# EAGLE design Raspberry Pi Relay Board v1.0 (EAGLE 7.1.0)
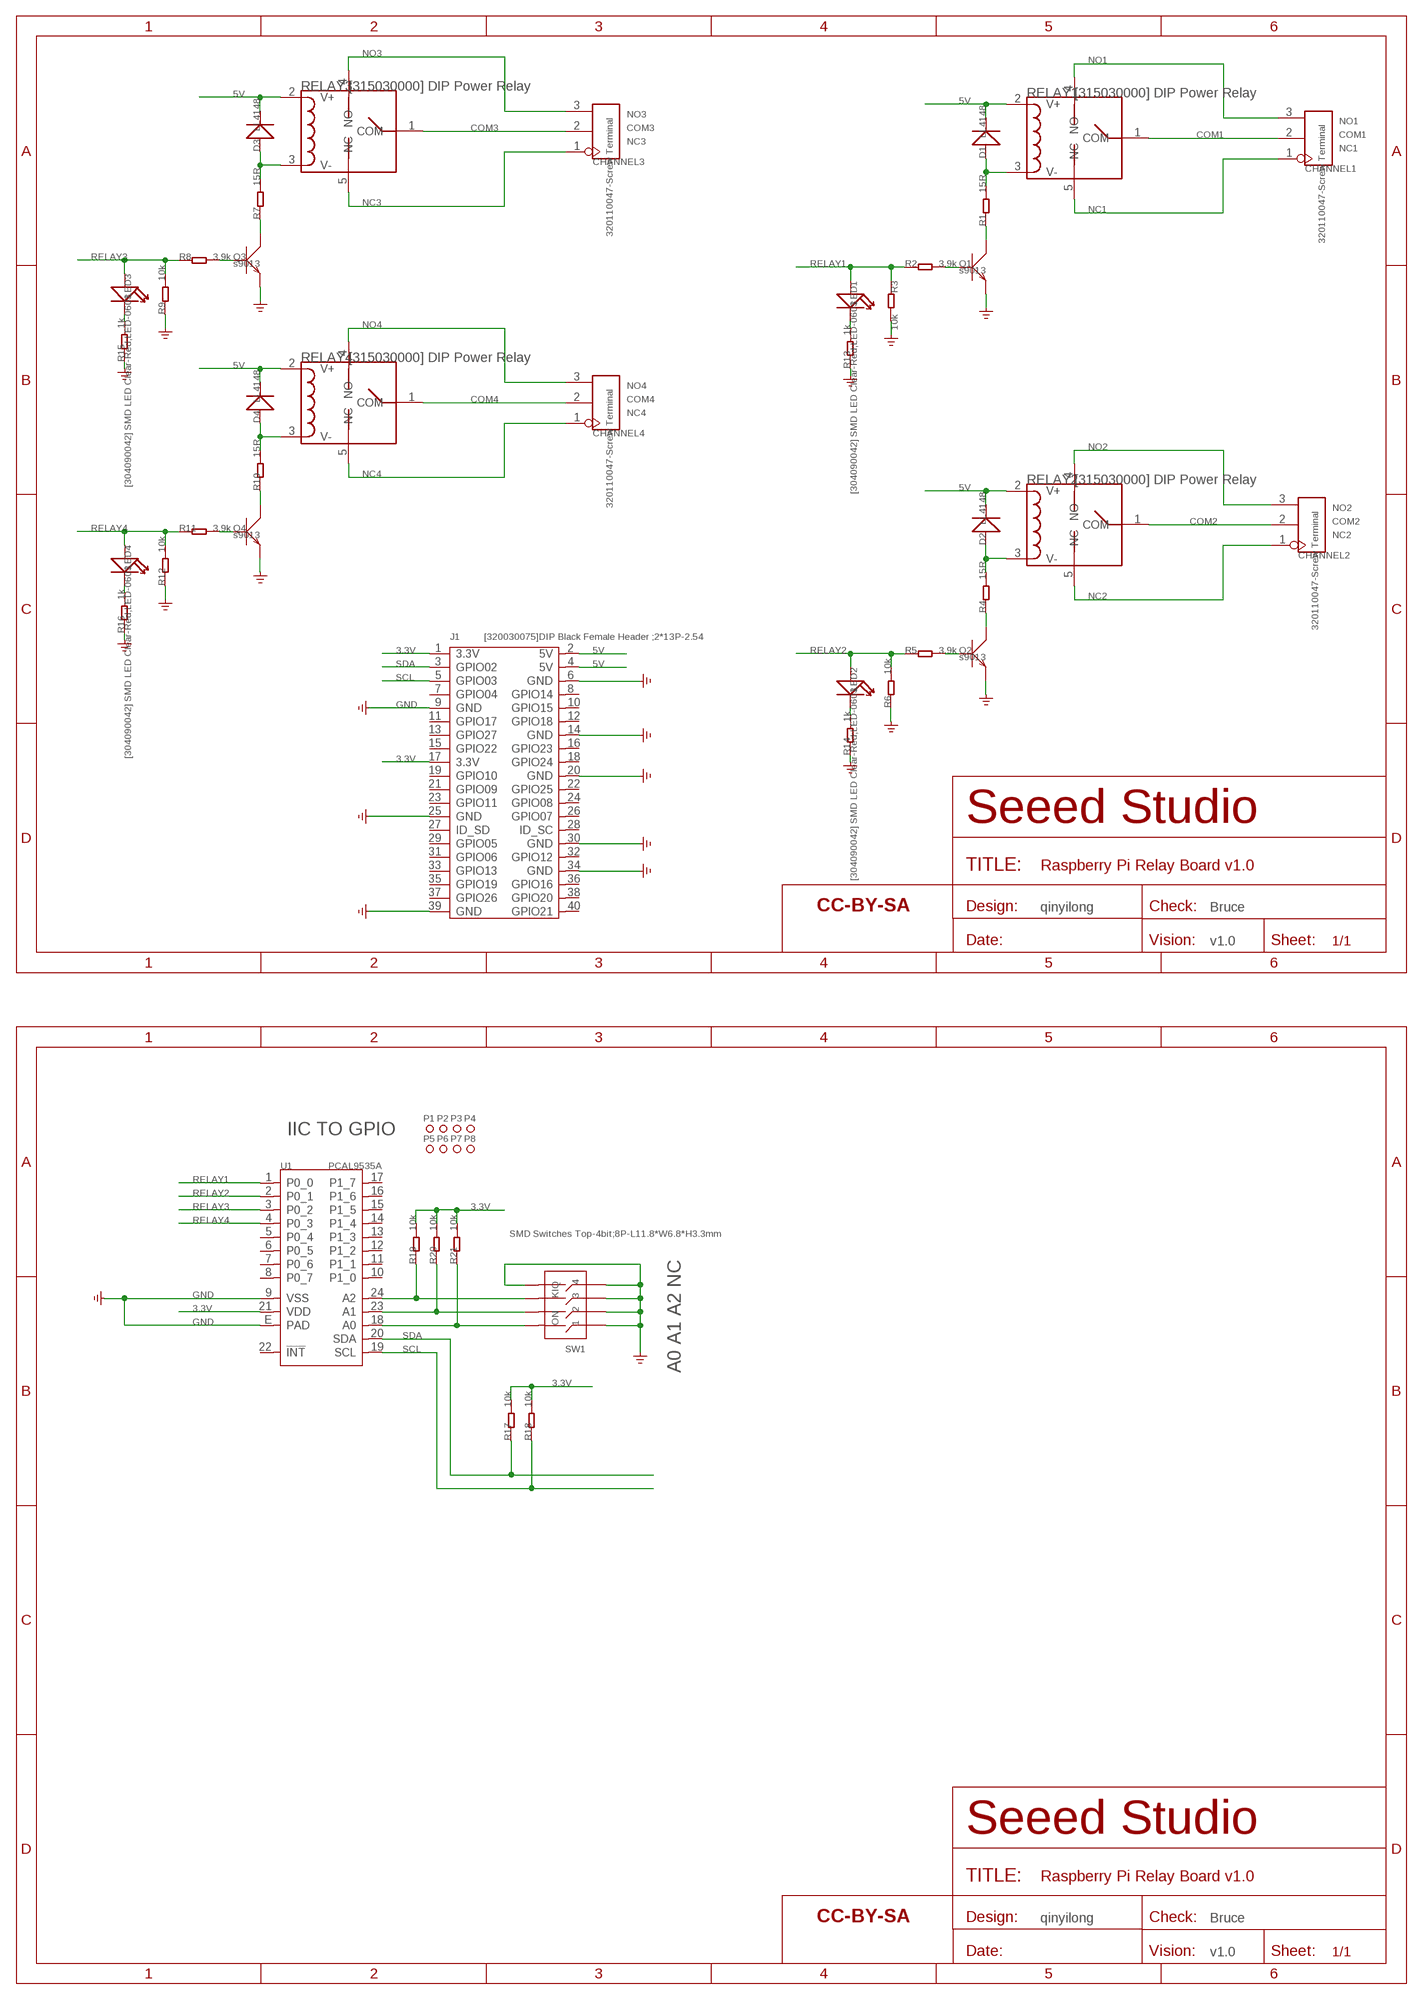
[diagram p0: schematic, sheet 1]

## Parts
CHANNEL1  320110047-Screw Terminal  SCREW-TERMINAL-3P'3.5'  [3P-3.5]
CHANNEL2  320110047-Screw Terminal  SCREW-TERMINAL-3P'3.5'  [3P-3.5]
CHANNEL3  320110047-Screw Terminal  SCREW-TERMINAL-3P'3.5'  [3P-3.5]
CHANNEL4  320110047-Screw Terminal  SCREW-TERMINAL-3P'3.5'  [3P-3.5]
D1  LL4148  D'1N4148-SMD'  [LL-34]
D2  LL4148  D'1N4148-SMD'  [LL-34]
D3  LL4148  D'1N4148-SMD'  [LL-34]
D4  LL4148  D'1N4148-SMD'  [LL-34]
J1  [320030075]DIP Black Female Header ;2*13P-2.54  HEADER-2X20P  [2X20P-2.54-65/35MIL]
LED1  [304090042] SMD LED Clear-Red;LED-0603  LED'0603'  [LED-0603]
LED2  [304090042] SMD LED Clear-Red;LED-0603  LED'0603'  [LED-0603]
LED3  [304090042] SMD LED Clear-Red;LED-0603  LED'0603'  [LED-0603]
LED4  [304090042] SMD LED Clear-Red;LED-0603  LED'0603'  [LED-0603]
P1  PAD-MARK'ANNULAR'  [ROUND-MARK-1.0]
P2  PAD-MARK'ANNULAR'  [ROUND-MARK-1.0]
P3  PAD-MARK'ANNULAR'  [ROUND-MARK-1.0]
P4  PAD-MARK'ANNULAR'  [ROUND-MARK-1.0]
P5  PAD-MARK'ANNULAR'  [ROUND-MARK-1.0]
P6  PAD-MARK'ANNULAR'  [ROUND-MARK-1.0]
P7  PAD-MARK'ANNULAR'  [ROUND-MARK-1.0]
P8  PAD-MARK'ANNULAR'  [ROUND-MARK-1.0]
Q1  s9013  TRANSISTOR-NPN-SOT23  [SOT23]
Q2  s9013  TRANSISTOR-NPN-SOT23  [SOT23]
Q3  s9013  TRANSISTOR-NPN-SOT23  [SOT23]
Q4  s9013  TRANSISTOR-NPN-SOT23  [SOT23]
R1  15R  R-0603  [R0603]
R2  3.9k  R-0603  [R0603]
R3  10k  R-0603  [R0603]
R4  15R  R-0603  [R0603]
R5  3.9k  R-0603  [R0603]
R6  10k  R-0603  [R0603]
R7  15R  R-0603  [R0603]
R8  3.9k  R-0603  [R0603]
R9  10k  R-0603  [R0603]
R10  15R  R-0603  [R0603]
R11  3.9k  R-0603  [R0603]
R12  10k  R-0603  [R0603]
R13  1k  R-0603  [R0603]
R14  1k  R-0603  [R0603]
R15  1k  R-0603  [R0603]
R16  1k  R-0603  [R0603]
R17  10k  R-0603  [R0603]
R18  10k  R-0603  [R0603]
R19  10k  R-0603  [R0603]
R20  10k  R-0603  [R0603]
R21  10k  R-0603  [R0603]
RELAY1  [315030000] DIP Power Relay  RELAY-HLS8L-DC5V-S-C  [5P-19.0X15.5X15.8H]
RELAY2  [315030000] DIP Power Relay  RELAY-HLS8L-DC5V-S-C  [5P-19.0X15.5X15.8H]
RELAY3  [315030000] DIP Power Relay  RELAY-HLS8L-DC5V-S-C  [5P-19.0X15.5X15.8H]
RELAY4  [315030000] DIP Power Relay  RELAY-HLS8L-DC5V-S-C  [5P-19.0X15.5X15.8H]
SW1  SMD Switches Top-4bit;8P-L11.8*W6.8*H3.3mm  SWITCHES-8P'KM-04'  [8P-SMD-L11.8*W6.8*H3.3MM]
U1  PCAL9535A  [QFN24]
U$23  SEEEDSTUDIO-OPEN-SCH-FRAME  [SEEEDSTUDIO-PCB-FRAME]
U$24  SEEEDSTUDIO-OPEN-SCH-FRAME  [SEEEDSTUDIO-PCB-FRAME]

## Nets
3.3V: J1.1(3.3V) J1.17(3.3V) R17.2 R18.2 R19.2 R20.2 R21.2 U1.21(VDD)
5V: D1.C(-) D2.C(-) D3.C(-) D4.C(-) J1.2(5V) J1.4(5V) RELAY1.2(V+) RELAY2.2(V+) RELAY3.2(V+) RELAY4.2(V+)
COM1: CHANNEL1.2 RELAY1.1(COM)
COM2: CHANNEL2.2 RELAY2.1(COM)
COM3: CHANNEL3.2 RELAY3.1(COM)
COM4: CHANNEL4.2 RELAY4.1(COM)
GND: J1.6(GND) J1.9(GND) J1.14(GND) J1.20(GND) J1.25(GND) J1.30(GND) J1.34(GND) J1.39(GND) Q1.2(E) Q2.2(E) Q3.2(E) Q4.2(E) R3.2 R6.1 R9.1 R12.1 R13.1 R14.1 R15.1 R16.1 SW1.1 SW1.2 SW1.3 SW1.4 SW1.5 U1.9(VSS) U1.E(PAD) ; supply symbol labelled GND_POWER
N$1: D2.A(+) R4.2 RELAY2.3(V-)
N$2: D3.A(+) R7.2 RELAY3.3(V-)
N$3: D4.A(+) R10.2 RELAY4.3(V-)
N$4: Q1.3(C) R1.1
N$5: Q2.3(C) R4.1
N$6: Q4.1(B) R11.2
N$7: D1.A(+) R1.2 RELAY1.3(V-)
N$8: Q3.3(C) R7.1
N$9: Q4.3(C) R10.1
N$11: Q3.1(B) R8.2
N$12: LED1.- R13.2
N$13: LED2.- R14.2
N$14: LED3.- R15.2
N$16: LED4.- R16.2
N$17: Q2.1(B) R5.2
N$23: Q1.1(B) R2.2
N$26: R19.1 SW1.6 U1.24(A2)
N$27: R20.1 SW1.7 U1.23(A1)
N$28: R21.1 SW1.8 U1.18(A0)
NC1: CHANNEL1.1 RELAY1.5(NC)
NC2: CHANNEL2.1 RELAY2.5(NC)
NC3: CHANNEL3.1 RELAY3.5(NC)
NC4: CHANNEL4.1 RELAY4.5(NC)
NO1: CHANNEL1.3 RELAY1.4(NO)
NO2: CHANNEL2.3 RELAY2.4(NO)
NO3: CHANNEL3.3 RELAY3.4(NO)
NO4: CHANNEL4.3 RELAY4.4(NO)
RELAY1: LED1.+ R2.1 R3.1 U1.1(P0_0)
RELAY2: LED2.+ R5.1 R6.2 U1.2(P0_1)
RELAY3: LED3.+ R8.1 R9.2 U1.3(P0_2)
RELAY4: LED4.+ R11.1 R12.2 U1.4(P0_3)
SCL: J1.5(GPIO03) R18.1 U1.19(SCL)
SDA: J1.3(GPIO02) R17.1 U1.20(SDA)
Unconnected: J1.7(GPIO04) J1.8(GPIO14) J1.10(GPIO15) J1.11(GPIO17) J1.12(GPIO18) J1.13(GPIO27) J1.15(GPIO22) J1.16(GPIO23) J1.18(GPIO24) J1.19(GPIO10) J1.21(GPIO09) J1.22(GPIO25) J1.23(GPIO11) J1.24(GPIO08) J1.26(GPIO07) J1.27(ID_SD) J1.28(ID_SC) J1.29(GPIO05) J1.31(GPIO06) J1.32(GPIO12) J1.33(GPIO13) J1.35(GPIO19) J1.36(GPIO16) J1.37(GPIO26) J1.38(GPIO20) J1.40(GPIO21) U1.5(P0_4) U1.6(P0_5) U1.7(P0_6) U1.8(P0_7) U1.10(P1_0) U1.11(P1_1) U1.12(P1_2) U1.13(P1_3) U1.14(P1_4) U1.15(P1_5) U1.16(P1_6) U1.17(P1_7) U1.22(!INT!)

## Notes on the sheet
- qinyilong | Bruce
- v1.0
- IIC TO GPIO
- A0 A1 A2 NC
- qinyilong | Bruce
- v1.0

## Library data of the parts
CHANNEL1-CHANNEL4 = Connector :SCREW-TERMINAL-3P
D1-D4 = Discrete:D*
J1 = Connector-new:HEADER-2X20P
LED1-LED4 = Discrete:LED*
P1-P8 = Discrete-new:PAD-MARK; PARTNO: DNP
Q1-Q4 = Discrete:TRANSISTOR-NPN*: NPN audion
R1-R21 = Discrete:R*
RELAY1-RELAY4 = Discrete:RELAY-HLS8L-DC5V-S-C
SW1 = Discrete-new:SWITCHES-8P: 311080003
U1 = template:PCAL9535A: Low-voltage 16-bit I2C-bus I/O port with interrupt and Agile I/O
U$23 U$24 = moudle-new:SEEEDSTUDIO-OPEN-SCH-FRAME

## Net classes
0 default: width 0.152 mm, drill 0.305 mm, clearance 0.152 mm

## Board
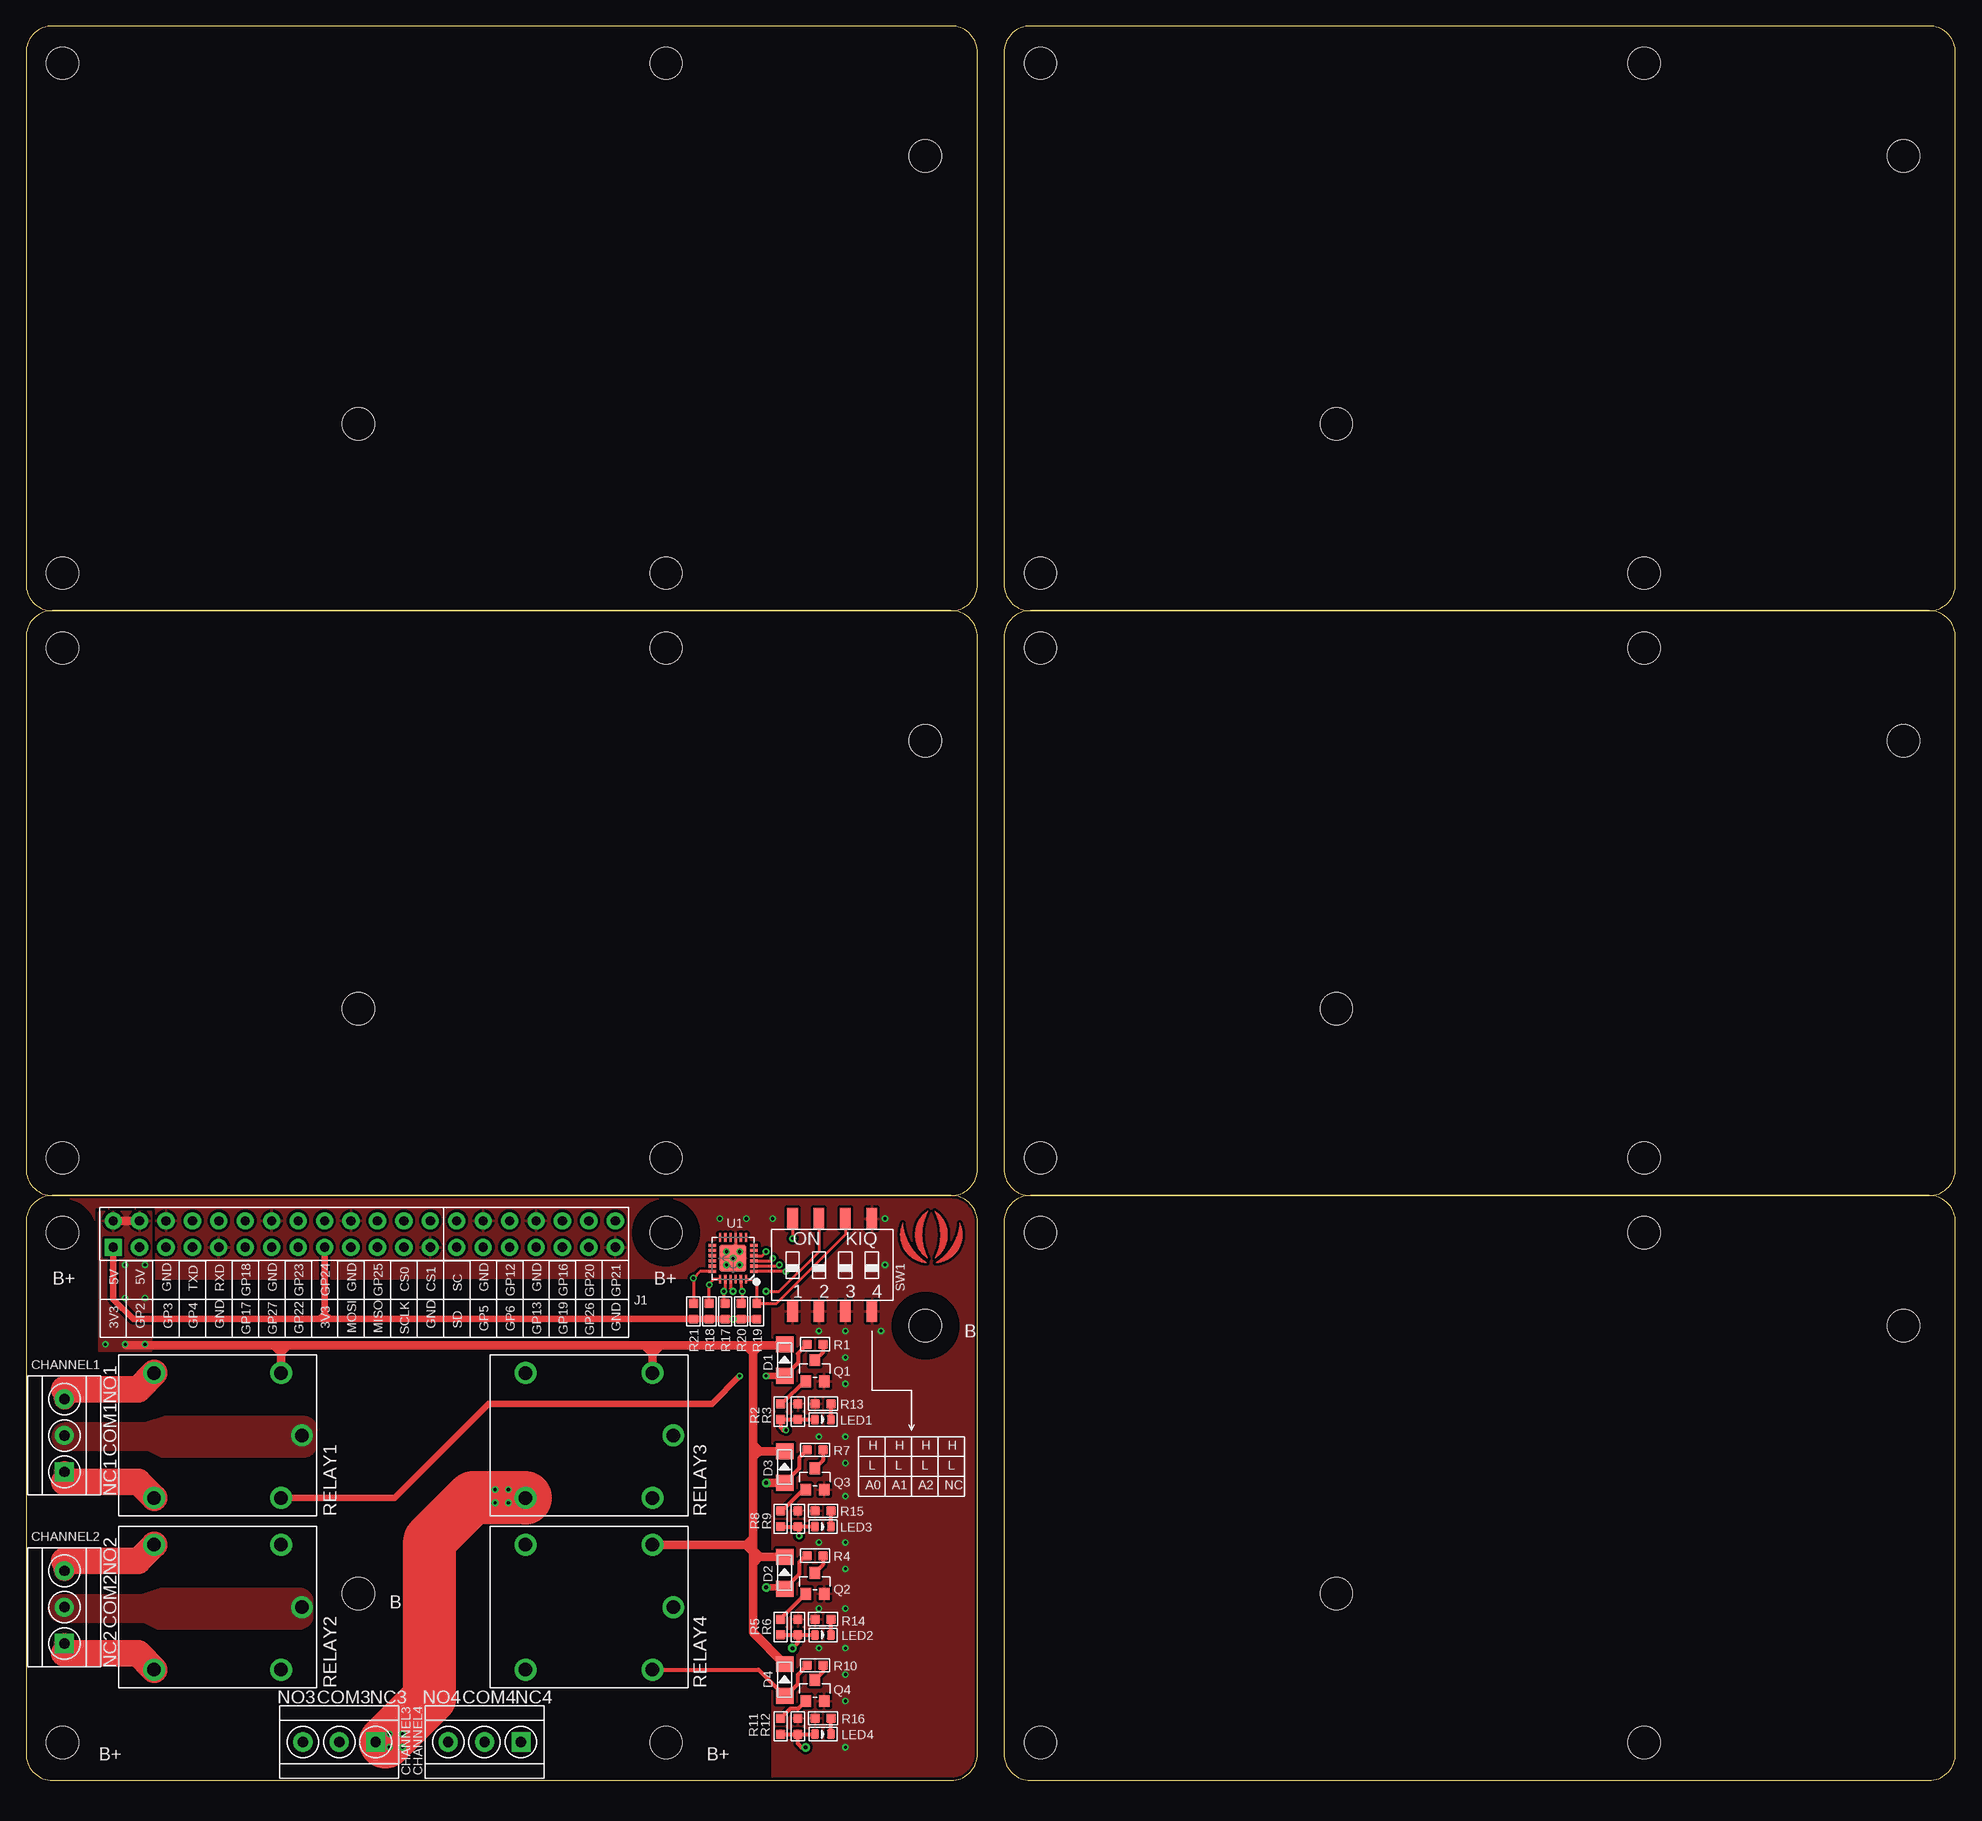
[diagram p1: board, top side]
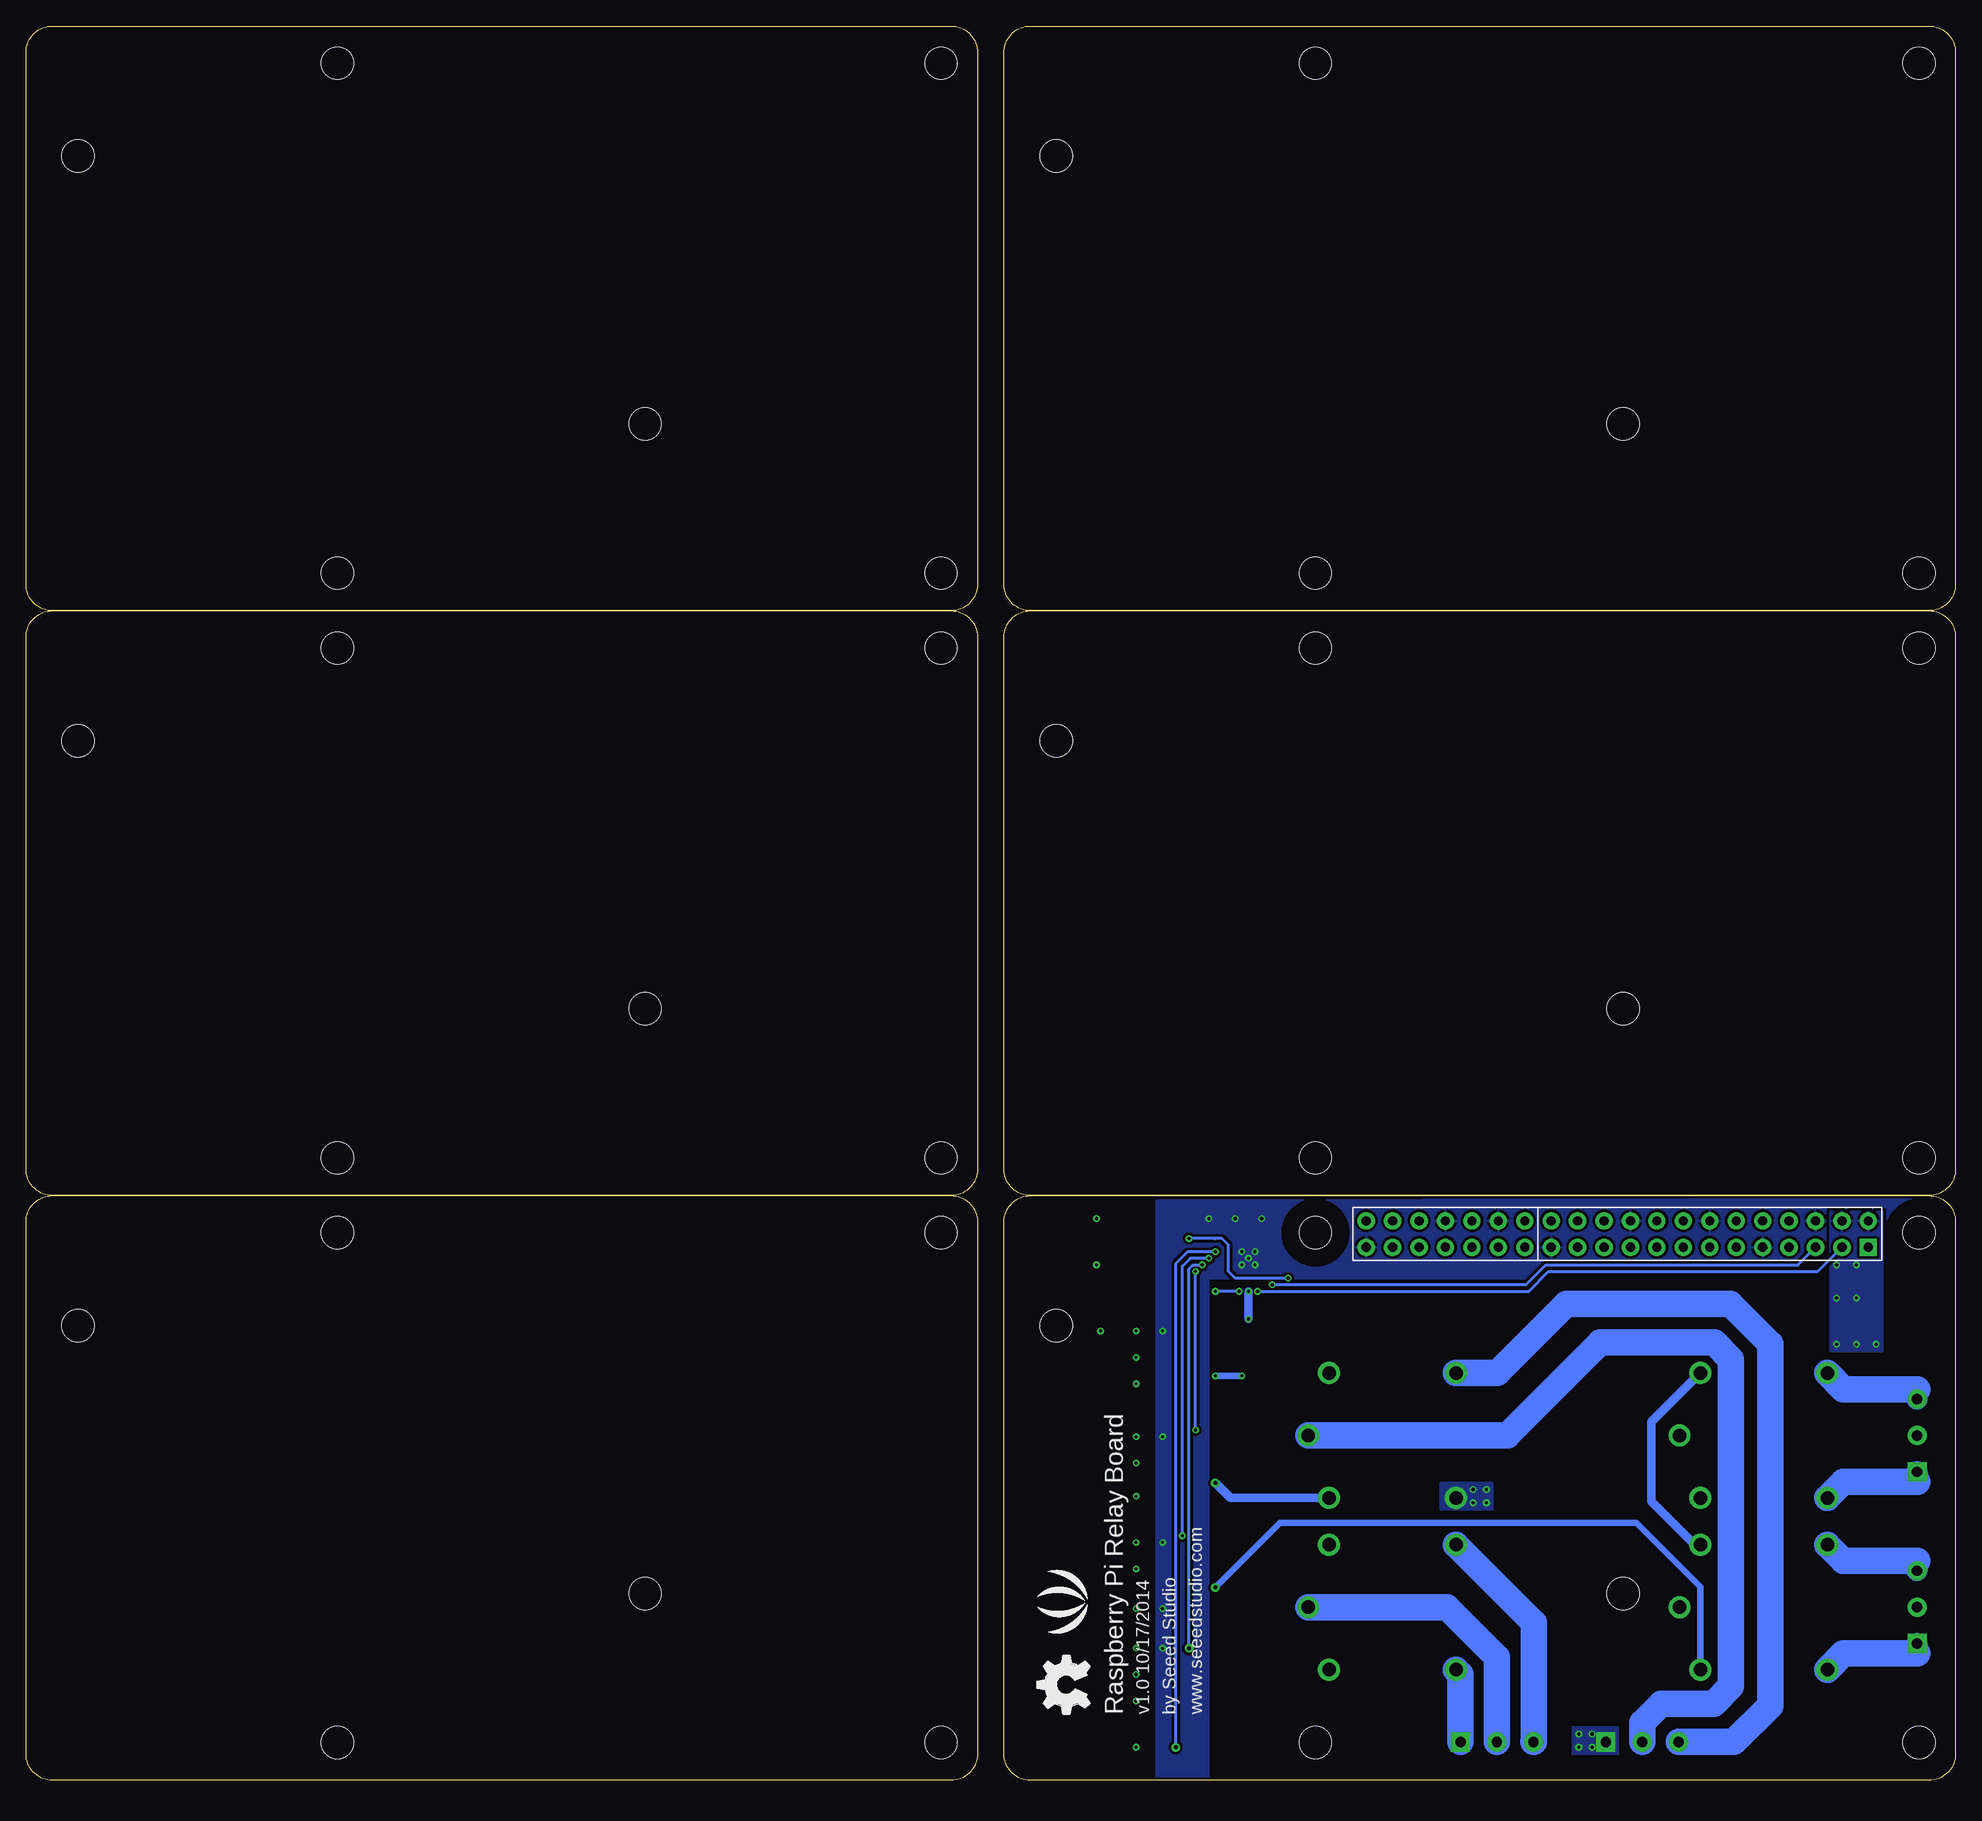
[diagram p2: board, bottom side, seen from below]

Size 185.42 x 168.59 mm. Coordinates in mm from the lower left corner, seen from the top.
Copper layers (1*16): Top 0.035mm / dielectric 1.5mm / Bottom 0.035mm
Design rules "default": minimum track width 6mil, minimum drill 12mil, track to track 6mil, track to pad 6mil, pad to pad 6mil, via to via 6mil, smd to smd 0mil, copper to edge 10mil, drill to drill 10mil, minimum pad ring 10mil, minimum via ring 6mil, stop-mask expansion 2mil, vias tented up to drill 100mil, thermal gap 10mil
Holes 2.03 mm at 2.54,173.35 182.88,173.35 182.88,-5.08 2.54,-5.08

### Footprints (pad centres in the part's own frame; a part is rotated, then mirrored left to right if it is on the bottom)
3P-3.5 = drill 1 pad 1.85 square: 1 0,-3.5 | drill 1 pad 1.85: 2 0,0; 3 0,3.5
LL-34 = smd 1.524 x 1.676: A -1.524,0; C 1.524,0
2X20P-2.54-65/35MIL = drill 0.889 pad 1.651 square: 1 1.27,24.13 | drill 0.889 pad 1.651: 2 -1.27,24.13; 3 1.27,21.59; 4 -1.27,21.59; 5 1.27,19.05; 6 -1.27,19.05; 7 1.27,16.51; 8 -1.27,16.51; 9 1.27,13.97; 10 -1.27,13.97; 11 1.27,11.43; 12 -1.27,11.43; 13 1.27,8.89; 14 -1.27,8.89; 15 1.27,6.35; 16 -1.27,6.35; 17 1.27,3.81; 18 -1.27,3.81; 19 1.27,1.27; 20 -1.27,1.27; 21 1.27,-1.27; 22 -1.27,-1.27; 23 1.27,-3.81; 24 -1.27,-3.81; 25 1.27,-6.35; 26 -1.27,-6.35; 27 1.27,-8.89; 28 -1.27,-8.89; 29 1.27,-11.43; 30 -1.27,-11.43; 31 1.27,-13.97; 32 -1.27,-13.97; 33 1.27,-16.51; 34 -1.27,-16.51; 35 1.27,-19.05; 36 -1.27,-19.05; 37 1.27,-21.59; 38 -1.27,-21.59; 39 1.27,-24.13; 40 -1.27,-24.13
LED-0603 = smd 0.762 x 0.889: + -0.762,0; - 0.762,0
ROUND-MARK-1.0 = smd 1.016 x 1.016: P$1 0,0
SOT23 = smd 1.016 x 1.143: 1 -0.889,-1.016; 2 0.889,-1.016; 3 0,1.016
R0603 = smd 0.889 x 0.889: 1 -0.762,0; 2 0.762,0
5P-19.0X15.5X15.8H = drill 1.3 pad 2.1: 1 -8.1,0; 2 -6.1,-6; 3 -6.1,6; 4 6.1,-6; 5 6.1,6
8P-SMD-L11.8*W6.8*H3.3MM = smd 1.016 x 2.032: 1 -3.81,-4.445; 2 -1.27,-4.445; 3 1.27,-4.445; 4 3.81,-4.445; 5 3.81,4.445; 6 1.27,4.445; 7 -1.27,4.445; 8 -3.81,4.445
QFN24 = smd 0.8 x 0.26: 1 -2,1.25; 2 -2,0.75; 3 -2,0.25; 4 -2,-0.25; 5 -2,-0.75; 6 -2,-1.25; 13 2,-1.25; 14 2,-0.75; 15 2,-0.25; 16 2,0.25; 17 2,0.75; 18 2,1.25 | smd 0.26 x 0.8: 7 -1.25,-2; 8 -0.75,-2; 9 -0.25,-2; 10 0.25,-2; 11 0.75,-2; 12 1.25,-2; 19 1.25,2; 20 0.75,2; 21 0.25,2; 22 -0.25,2; 23 -0.75,2; 24 -1.25,2 | smd 2.6 x 2.6: E 0.02,-0.01
RASPBERRY-PI-B+/B = hole 3.1: 3.503,52.622; 3.503,3.622; 61.503,52.622; 61.503,3.622; 31.951,17.951; 86.431,43.7

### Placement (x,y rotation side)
CHANNEL1  3.68,33.15 0 top
CHANNEL2  3.68,16.64 0 top
CHANNEL3  30.1,3.68 90 top
CHANNEL4  44.07,3.68 90 top
D1  72.9,40.39 90 top
D2  72.9,19.94 90 top
D3  72.9,30.1 90 top
D4  72.9,9.65 90 top
J1  32.5,52.5 270 bottom
LED1  76.58,34.67 0 top
LED2  76.58,13.97 0 top
LED3  76.58,24.38 0 top
LED4  76.58,4.45 0 top
P1  not placed on the board
P2  not placed on the board
P3  not placed on the board
P4  not placed on the board
P5  not placed on the board
P6  not placed on the board
P7  not placed on the board
P8  not placed on the board
Q1  75.82,39.37 0 top
Q2  75.82,18.92 0 top
Q3  75.82,28.96 0 top
Q4  75.82,8.64 0 top
R1  75.82,41.91 180 top
R2  72.52,35.43 90 top
R3  74.17,35.43 90 top
R4  75.82,21.59 180 top
R5  72.52,14.73 90 top
R6  74.17,14.73 270 top
R7  75.82,31.75 180 top
R8  72.52,25.15 90 top
R9  74.17,25.15 270 top
R10  75.82,11.05 180 top
R11  72.52,5.21 90 top
R12  74.17,5.21 270 top
R13  76.58,36.2 0 top
R14  76.58,15.49 0 top
R15  76.58,25.91 0 top
R16  76.58,5.97 0 top
R17  67.18,45.09 270 top
R18  65.66,45.09 270 top
R19  70.23,45.09 270 top
R20  68.71,45.09 270 top
R21  64.14,45.09 270 top
RELAY1  18.41,33.15 180 top
RELAY2  18.41,16.64 180 top
RELAY3  54.1,33.15 180 top
RELAY4  54.1,16.64 180 top
SW1  77.47,49.53 0 top
U1  67.94,50.16 180 top
U$13  [LOGO_SILK]  85.09,17.14 90 bottom
U$14  [OSHW_FILLX200_NOTEXT]  83.19,6.35 90 bottom
U$23  not placed on the board
U$24  not placed on the board
U$27  [RASPBERRY-PI-B+/B]  0,0 0 top
U$28  [SEEED-COPPER-280*268MIL]  87,51.44 0 top
U$29  [RASPBERRY-PI-B+/B]  0,56.2 0 top
U$30  [RASPBERRY-PI-B+/B]  0,112.39 0 top
U$31  [RASPBERRY-PI-B+/B]  93.98,0 0 top
U$32  [RASPBERRY-PI-B+/B]  93.98,56.2 0 top
U$33  [RASPBERRY-PI-B+/B]  93.98,112.39 0 top

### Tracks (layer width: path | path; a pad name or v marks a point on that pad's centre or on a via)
3.3V  (via drill 0.3 pad 0.64)
  Top 0.305: U1.21 67.69,47.24 v67.94,46.99
  Top 0.61: 29.21,44.32 R21.2 R18.2 R17.2 v67.94,44.32 R20.2 R19.2 | 29.21,44.32 28.7,44.32 | 28.19,44.32 10.29,44.32 8.37,46.24 J1.1 | J1.17 28.69,44.83 | 28.69,44.82 28.69,44.34 28.7,44.32 | 28.69,44.83 28.7,44.83 29.21,44.32 | 28.69,44.83 28.69,44.82 | 28.69,44.82 28.19,44.32 | 28.19,44.32 28.7,44.32
  Bottom 0.813: v67.94,46.99 v67.94,44.32
5V  (via drill 0.3 pad 0.64)
  Top 0.813: D1.C 72.77,41.78 69.85,41.78 | J1.4 J1.2 | 69.85,41.78 69.22,41.78 | 69.22,41.78 60.2,41.78 | 60.2,41.78 59.44,41.78 | 59.44,41.78 24.51,41.78 | 24.51,41.78 9.65,41.78 | RELAY3.2 60.2,41.78 | D3.C 70.48,31.62 | 70.48,31.62 69.85,31.62 | 69.85,31.62 69.85,23.24 | 69.85,23.24 69.85,22.73 | 69.85,22.73 69.85,22.1 | 69.85,22.1 69.85,21.46 | 69.85,21.46 69.85,20.83 | 69.85,20.83 69.85,14.22 D4.C | D2.C 70.48,21.46 | 70.48,21.46 69.85,21.46 | RELAY4.2 69.18,22.64 | 69.25,22.64 69.75,22.64 69.85,22.73 | 69.85,31.62 69.85,41.78 | RELAY1.2 24.52,41.14 | 24.52,41.15 24.52,41.78 24.51,41.78 | 24.52,41.14 24,41.66 | 24.52,41.14 24.52,41.15 | 24.52,41.15 25.02,41.66 | 59.44,41.78 60.2,41.02 60.83,41.66 | 69.22,41.78 69.72,41.27 69.98,41.27 70.36,41.66 | 70.48,31.62 69.98,32.13 | 70.48,31.62 69.98,31.11 | 69.18,22.64 69.25,22.64 | 69.25,22.64 69.85,23.24 | 69.18,22.64 69.72,22.1 | 70.48,21.46 69.85,22.1 | 70.48,21.46 69.85,20.83
  Bottom 0.813: RELAY2.2 25.05,22.64 29.21,26.8 29.21,34.45 RELAY1.2
  other vias: 7.62,41.91 9.53,41.91 11.43,41.91 11.43,46.35 9.53,46.35 9.53,49.53 11.43,49.53
  pour Bottom (isolate 0.254): 6.99,54.61 12.06,54.61 12.06,41.27 6.99,41.27
  pour Top (isolate 0.254): 12.06,54.61 6.99,54.61 6.99,41.27 12.06,41.27
COM1
  pour Top (isolate 0.254, no thermals): 11.43,34.29 3.81,34.29 arc90 2.54,33.02 arc90 3.81,31.75 11.68,31.75 12.95,31.11 26.67,31.11 arc90 27.94,32.38 27.94,33.66 arc90 26.67,34.92 13.34,34.92
COM2
  pour Top (isolate 0.254, no thermals): 11.05,17.78 3.43,17.78 arc90 2.16,16.51 arc90 3.43,15.24 11.3,15.24 12.57,14.61 26.29,14.61 arc90 27.56,15.88 27.56,17.14 arc90 26.29,18.41 12.95,18.41
COM3
  Bottom 2.54: RELAY3.1 43.05,33.15 34.12,42.08 23.2,42.08 21.59,40.47 21.59,9.02 23.24,7.37 28.27,7.37 30.1,5.53 CHANNEL3.2
COM4
  Bottom 2.54: RELAY4.1 48.9,16.64 44.07,11.81 CHANNEL4.2
GND  (via drill 0.3 pad 0.64)
  Top 0.203: 76.77,7.43 76.71,7.43 Q4.2 | 76.77,17.91 76.77,17.71
  Top 0.305: U1.9 68.19,50.45 U1.E
  other vias: 67.31,50.8 68.58,50.8 68.58,49.53 67.31,49.53 67.94,50.16 76.2,43.18 78.74,43.18 78.74,40.64 78.74,38.1 78.74,7.62 78.74,10.16 78.74,12.7 78.74,16.51 78.74,20.32 78.74,22.86 78.74,27.3 78.74,30.48 78.74,33.02 76.2,12.7 76.2,16.51 76.2,22.86 76.2,33.02 78.74,3.17 82.17,43.18 82.55,53.98 82.55,49.53 71.75,53.98 69.22,53.98 66.67,53.98
  pour Top (isolate 0.254, rank 6): 0,55.88 91.44,55.88 91.44,0 71.75,0 71.75,48.26 0,48.13
  pour Bottom (isolate 0.254, rank 6): 0,55.88 76.83,55.75 76.83,-0.13 71.75,0 71.75,48.26 0,48.26
N$1  (via drill 0.38 pad 0.81)
  Top 0.406: R4.2 74.93,21.59 74.3,20.95 74.3,19.81 D2.A
  Top 0.61: v71.12,18.54 72.77,18.54 D2.A
  Bottom 0.61: RELAY2.3 24.52,18.62 30.66,24.77 64.9,24.77 v71.12,18.54
N$2  (via drill 0.38 pad 0.81)
  Top 0.406: R7.2 74.3,30.99 74.3,29.97 D3.A
  Top 0.813: D3.A v71.12,28.57
  Bottom 0.813: RELAY3.3 69.69,27.15 v71.12,28.57
N$3
  Top 0.406: R10.2 74.17,10.16 74.17,9.27 73.41,8.51 73.41,8 73.28,8.13 D4.A 70.39,10.64 RELAY4.3
N$4
  Top 0.406: R1.1 76.58,41.15 Q1.3
N$5
  Top 0.406: R4.1 76.58,20.7 Q2.3
N$6
  Top 0.406: Q4.1 74.17,6.86 73.41,6.86 R11.2
N$7  (via drill 0.3 pad 0.64)
  Top 0.406: R1.2 74.17,41.02 74.17,40.13 D1.A
  Top 0.61: 27.66,27.15 RELAY1.3 35.4,27.15 44.45,36.2 65.91,36.2 v68.58,38.86 | 72.39,38.86 D1.A v71.12,38.86
  Bottom 0.61: v68.58,38.86 v71.12,38.86
N$8
  Top 0.406: R7.1 76.58,30.73 Q3.3
N$9
  Top 0.406: R10.1 76.58,10.41 Q4.3
N$11
  Top 0.406: R8.2 72.64,25.91 74.68,27.94 Q3.1
N$12
  Top 0.406: LED1.- R13.2
N$13
  Top 0.406: LED2.- R14.2
N$14
  Top 0.406: LED3.- R15.2
N$16
  Top 0.406: LED4.- R16.2
N$17
  Top 0.406: R5.2 72.52,15.55 72.58,15.55 Q2.1
N$23
  Top 0.406: R2.2 72.71,36.2 72.71,36.26 74.8,38.35 Q1.1
N$26
  Top 0.305: SW1.6 78.74,52.45 72.14,45.85 R19.1 70.23,47.75 69.82,48.16 U1.24
N$27  (via drill 0.3 pad 0.64)
  Top 0.305: 68.44,46.11 R20.1 | SW1.7 76.2,50.8 72.39,46.99 v71.12,46.99 | 68.5,45.8 68.58,45.72 R20.1 | 68.82,45.96 R20.1 | R20.1 68.83,45.97 v68.83,46.99 68.69,47.13 U1.23
  Bottom 0.305: v68.83,46.99 v71.12,46.99
N$28  (via drill 0.3 pad 0.64)
  Top 0.305: U1.18 64.79,48.91 v64.14,48.26 R21.1 | SW1.8 v73.66,52.07
  Bottom 0.305: v73.66,52.07 71.25,52.07 71.12,52.07 70.48,52.07 69.85,51.44 69.85,48.9 69.22,48.26 v64.14,48.26
NC1
  Top 2.032: CHANNEL1.1 3.68,28.7
  Top 2.54: 3.68,28.7 10.76,28.7 RELAY1.5
  Bottom 2.032: CHANNEL1.1 3.68,28.7
  Bottom 2.54: 3.68,28.7 10.76,28.7 RELAY1.5
NC2
  Top 2.032: CHANNEL2.1 3.68,12.19
  Top 2.54: 3.68,12.19 10.76,12.19 RELAY2.5
  Bottom 2.032: CHANNEL2.1 3.68,12.19
  Bottom 2.54: 3.68,12.19 10.76,12.19 RELAY2.5
NC3  (via drill 0.3 pad 0.64)
  Top 2.54: CHANNEL3.1 34.54,3.68
  Top 5.08: RELAY3.5 47.97,27.18 42.93,27.18 38.8,23.05 38.8,7.94 34.54,3.68
  other vias: 46.35,26.67 46.35,27.94 45.09,27.94 45.09,26.67 34.92,4.45 36.2,4.45 36.2,3.17 34.92,3.17
  pour Bottom (isolate 0.254, no thermals): 44.45,28.57 49.53,28.57 49.53,26.04 44.45,26.04
  pour Bottom (isolate 0.254, no thermals): 32.38,2.54 32.38,5.08 36.83,5.08 36.83,2.54
NC4
  Bottom 2.54: CHANNEL4.1 47.57,10.2 RELAY4.5
NO1
  Top 2.032: CHANNEL1.3 3.68,37.59
  Top 2.54: 3.68,37.59 10.76,37.59 RELAY1.4
  Bottom 2.032: CHANNEL1.3 3.68,37.59
  Bottom 2.54: 3.68,37.59 10.76,37.59 RELAY1.4
NO2
  Top 2.032: CHANNEL2.3 3.68,21.08
  Top 2.54: 3.68,21.08 10.76,21.08 RELAY2.4
  Bottom 2.032: 3.68,21.08 CHANNEL2.3
  Bottom 2.54: 3.68,21.08 10.76,21.08 RELAY2.4
NO3
  Bottom 2.54: CHANNEL3.3 21.28,3.68 17.78,7.19 17.78,41.94 21.63,45.79 37.4,45.79 44.04,39.15 RELAY3.4
NO4
  Bottom 2.54: CHANNEL4.3 40.51,3.68 40.51,15.15 RELAY4.4
RELAY1  (via drill 0.3 pad 0.64)
  Top 0.305: v73.03,48.9 69.97,48.9 U1.1
  Top 0.406: R2.1 R3.1 LED1.+ | 72.39,34.54 R2.1 | R2.1 72.52,33.91 72.77,33.66 v73.03,33.66
  Bottom 0.305: v73.03,33.66 v73.03,48.9
RELAY2  (via drill 0.3 pad 0.64, 0.38 pad 0.81)
  Top 0.305: 72.33,49.47 v72.39,49.53 72.28,49.41 U1.2
  Top 0.406: R5.1 R6.2 | R6.2 LED2.+ | R6.2 74.17,13.21 v73.66,12.7
  Bottom 0.305: v73.66,12.7 73.66,49.15 73.28,49.53 v72.39,49.53
RELAY3  (via drill 0.3 pad 0.64)
  Top 0.305: 71.63,50.04 v71.75,50.16 71.5,49.91 U1.3
  Top 0.406: R8.1 R9.2 74.3,24.38 | LED3.+ 74.3,24.38 | v74.3,23.5 74.3,24.38
  Bottom 0.305: v71.75,50.16 73.53,50.16 74.3,49.4 v74.3,23.5
RELAY4  (via drill 0.3 pad 0.64, 0.38 pad 0.81)
  Top 0.305: U1.4 70.73,50.41 v71.12,50.8
  Top 0.406: R11.1 R12.2 | R12.2 LED4.+ | v74.93,3.17 74.53,3.17 74.17,3.53 R12.2
  Bottom 0.305: v71.12,50.8 73.79,50.8 74.93,49.66 v74.93,3.17
SCL  (via drill 0.3 pad 0.64)
  Top 0.305: R18.1 65.66,47.37 v65.66,47.62 65.66,47.75 66.07,48.16 U1.19
  Bottom 0.305: J1.5 15.15,49.53 39.37,49.53 41.27,47.62 v65.66,47.62
SDA  (via drill 0.3 pad 0.64)
  Top 0.305: U1.20 67.19,47.13 v67.06,46.99 67.06,45.97 R17.1
  Bottom 0.305: J1.3 13.24,48.9 39.12,48.9 41.02,46.99 v67.06,46.99

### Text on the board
tPlace: B+ | 5V | 5V | B+ | GND | TXD | RXD | GP18 | GND | GP23 | GP24 | GND | GP25 | CS0 | CS1 | SC | GND | GP12 | GND | GP16 | GP20 | GP21 | 3V3 | GP2 | GP3 | GP4 | GND | GP17 | GP27 | GP22 | 3V3 | MOSI | MISO | SCLK | GND | SD | GP5 | GP6 | GP13 | GP19 | GP26 | GND | B | NO1 | H | H | H | H | COM1 | L | L | L | L | A0 | A1 | A2 | NC | NC1 | NO2 | B | COM2 | NC2 | NO3 | COM3 | NC3 | NO4 | COM4 | NC4 | B+ | B+
bPlace: www.seeedstudio.com | by Seeed Studio | v1.0 10/17/2014 | Raspberry Pi Relay Board

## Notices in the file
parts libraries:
moudle-new: This work is licensed under the Creative Commons Attribution 4.0 International License.
To view a copy of this license,visit:
http://creativecommons.org/licenses/by-sa/4.0
moudle-new: CC-BY-SA
